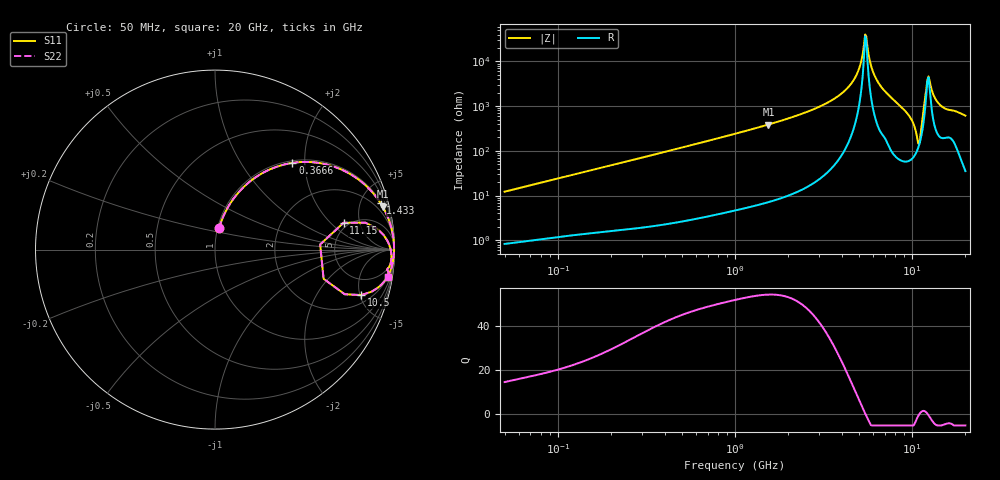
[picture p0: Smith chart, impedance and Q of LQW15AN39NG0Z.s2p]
!Murata Part Number: LQW15AN39NG0Z
!These Parameters are Measured in Series Mode Connection
!  o--[Z]--o
!Port1  Port2
!  o-------o
!Freq. Start=50[MHz] Stop=20[GHz], 401[Steps]
# Hz S RI R 50
!Freq.(Hz) S11(Real) S11(Imag) S21(Real) S21(Imag) S12(Real) S12(Imag) S22(Real) S22(Imag)
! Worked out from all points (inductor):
!   401 points, 50 MHz to 20 GHz, reference 50 ohm
!   read as one part in series: L = 38.6 nH near 51.52 MHz
!   highest Q = 54.4 at 1.544 GHz (marker M1), where L = 40 nH
!   self-resonance near 5.434 GHz
!   S11 on the Smith chart (normalised r, x): 50 MHz: 1.02, +0.24; 366.6 MHz: 1.04, +1.73; 1.433 GHz: 1.13, +7.13; 10.5 GHz: 2.76, -5.16; 11.15 GHz: 4.52, +2.90; 20 GHz: 2, -12
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5e7  0.0225 0.1183  0.9775 -0.1183  0.9775 -0.1183  0.0225 0.1183
1.364002e8  0.1058 0.2873  0.8942 -0.2873  0.8942 -0.2873  0.1058 0.2873
3.665683e8  0.4309 0.483  0.5691 -0.483  0.5691 -0.483  0.4309 0.483
3.721004e8  0.4381 0.484  0.5619 -0.484  0.5619 -0.484  0.4381 0.484
1e9  0.8483 0.3492  0.1517 -0.3492  0.1517 -0.3492  0.8483 0.3492
1.432596e9  0.9229 0.2576  0.0771 -0.2576  0.0771 -0.2576  0.9229 0.2576
1.544007e9  0.9339 0.2394  0.0661 -0.2394  0.0661 -0.2394  0.9339 0.2394
2.728004e9  0.9831 0.1183  0.0169 -0.1183  0.0169 -0.1183  0.9831 0.1183
4.472136e9  0.9968 0.0333  0.00324 -0.0333  0.00324 -0.0333  0.9968 0.0333
4.966507e9  0.9976 0.016  0.00243 -0.016  0.00243 -0.016  0.9976 0.016
5.433528e9  0.9977 0.000996  0.00228 -0.000996  0.00228 -0.000996  0.9977 0.000996
5.598765e9  0.9976 -0.00412  0.00235 0.00412  0.00235 0.00412  0.9976 -0.00412
5.856089e9  0.9974 -0.0119  0.00259 0.0119  0.00259 0.0119  0.9974 -0.0119
6.217679e9  0.9968 -0.0227  0.00322 0.0227  0.00322 0.0227  0.9968 -0.0227
7.442007e9  0.9926 -0.0576  0.00739 0.0576  0.00739 0.0576  0.9926 -0.0576
9.745021e9  0.9527 -0.1644  0.0473 0.1644  0.0473 0.1644  0.9527 -0.1644
1.050288e10  0.8154 -0.2533  0.1846 0.2533  0.1846 0.2533  0.8154 -0.2533
1.115139e10  0.7162 0.1494  0.2838 -0.1494  0.2838 -0.1494  0.7162 0.1494
1.201863e10  0.9703 0.0276  0.0297 -0.0276  0.0297 -0.0276  0.9703 0.0276
1.238412e10  0.98 -0.00681  0.02 0.00681  0.02 0.00681  0.98 -0.00681
1.460232e10  0.9722 -0.0928  0.0278 0.0928  0.0278 0.0928  0.9722 -0.0928
2e10  0.9657 -0.1553  0.0343 0.1553  0.0343 0.1553  0.9657 -0.1553
